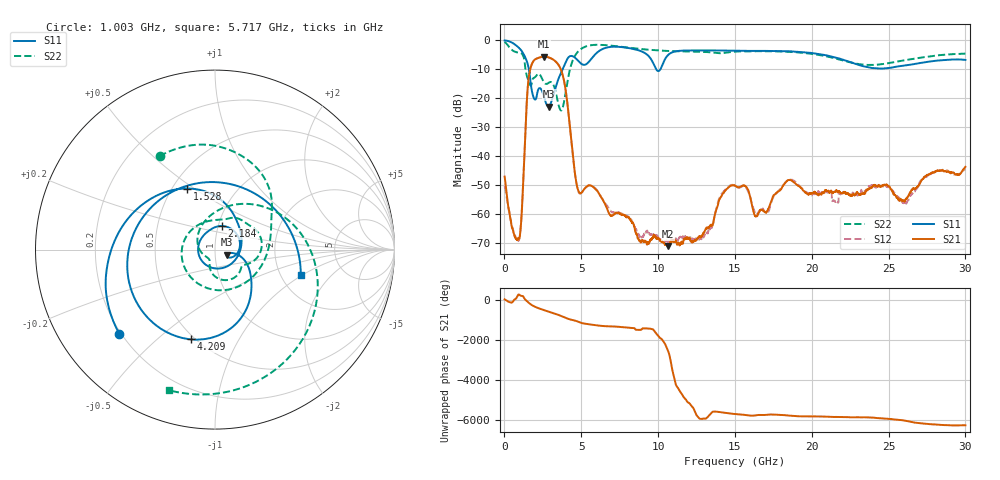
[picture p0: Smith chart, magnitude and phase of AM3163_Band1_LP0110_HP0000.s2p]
!Agilent Technologies,E8364B,MY43040894,A.07.50.67
!Agilent E8364B: A.07.50.67
!Date: Thursday, August 20, 2020 11:25:26
!Correction: S11(Full 2 Port(1,2))
!S21(Full 2 Port(1,2))
!S12(Full 2 Port(1,2))
!S22(Full 2 Port(1,2))
!S2P File: Measurements: S11, S21, S12, S22:
# Hz S  dB  R 50
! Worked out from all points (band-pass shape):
!   3201 points, 10 MHz to 30 GHz, reference 50 ohm
!   highest |S21| = -5.66 dB at 2.569 GHz (marker M1); lowest = -71.2 dB at 10.64 GHz (marker M2)
!   |S21| within 3 dB of the highest: 1.753 GHz to 3.534 GHz (1.78 GHz wide, 67.3 % of centre)
!   lowest |S11| = -22.9 dB at 2.868 GHz (marker M3), VSWR 1.15, Z = 56.9 - j3.32 ohm
!   |S11| at or under -10 dB: 1.589 GHz to 3.788 GHz (2.199 GHz wide, 81.8 % of centre); 9.869 GHz to 10.15 GHz (284.7 MHz wide, 2.84 % of centre)
!   |S22| runs from -24.3 to -0.6 dB; largest |S21 - S12| = 0.0074
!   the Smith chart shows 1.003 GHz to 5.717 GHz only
!   S11 on the Smith chart (normalised r, x): 1.003 GHz: 0.19, -0.37; 1.528 GHz: 0.60, +0.47; 2.184 GHz: 1.04, +0.28; 4.209 GHz: 0.48, -0.65; 5.717 GHz: 2.57, -0.97
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1e7  -0.09 -8.9  -47.14 48.9  -50.47 -122.0  -0.60 -24.6
5.254531e8  -0.95 -70.0  -65.00 -84.6  -64.85 -61.0  -3.53 -149.2
1.003419e9  -2.97 -138.6  -67.61 -96.5  -67.68 174.4  -4.36 120.7
1.528244e9  -8.56 114.2  -15.53 -90.3  -15.52 -90.4  -13.49 -116.6
1.884375e9  -19.61 -91.2  -7.23 76.2  -7.23 76.2  -13.13 48.8
2.184275e9  -17.27 73.3  -6.17 -26.7  -6.16 -26.7  -11.62 16.1
2.568522e9  -19.48 -23.2  -5.66 -131.0  -5.67 -131.1  -14.50 -26.3
2.868422e9  -22.93 -24.0  -5.93 154.2  -5.94 154.1  -14.76 -39.4
3.411991e9  -14.85 -21.0  -7.80 16.9  -7.81 16.9  -19.83 -106.6
4.2086e9  -5.72 -105.1  -27.31 135.7  -27.29 135.7  -11.30 66.8
5.014581e9  -8.21 114.0  -52.68 -55.3  -52.68 -55.4  -2.92 -51.0
5.717472e9  -6.04 -16.6  -50.48 -145.6  -50.40 -147.1  -1.68 -108.1
6.467222e9  -2.86 -99.4  -55.78 148.0  -55.67 147.5  -1.66 -153.0
7.479384e9  -2.31 -169.5  -59.88 111.4  -59.55 107.5  -2.20 158.8
1.000979e10  -10.67 89.8  -68.40 21.8  -68.21 -48.1  -3.54 59.9
1.063771e10  -5.18 88.7  -71.18 17.1  -69.65 177.9  -3.72 37.3
1.245585e10  -3.53 5.4  -69.03 84.0  -68.84 155.9  -3.96 -23.7
1.5005e10  -3.63 -72.3  -50.29 67.1  -50.26 68.0  -3.95 -90.5
2.000958e10  -4.43 163.1  -52.81 -55.3  -53.46 -58.6  -4.71 136.3
2.275554e10  -8.02 59.9  -53.30 -95.1  -53.15 -95.8  -7.97 20.8
2.500479e10  -9.61 -62.2  -50.55 -169.8  -50.55 -170.8  -7.95 -92.3
3e10  -6.83 104.0  -43.78 -135.0  -44.54 -134.7  -4.64 101.9
